| IBIS File
| Lattice Semiconductor Corporation
|[Doc Num]   FPGA-MD-02066 Ver. 1.0
[IBIS Ver]   4.2
[File name]   lifmd.ibs
[File rev]   2.5
[Date]   Mon May  6 22:10:33 PDT 2024
[Source]   Lattice Semiconductor umc40lp Process
[Notes]   Device: LIF-MD6000   Final
   Device: LIA-MD6000   Final
   Lattice Semiconductor has worked hard to ensure the
   models below are accurate and complete.  However, the
   data below was generated using simulation of the
   input/output model files for the silicon.  Therefore,
   the data below is for reference and initial design
   purposes only.
   Lattice Semiconductor grants permission to use this
   data for use in printed circuit design using this
   Lattice programmable logic device.  Other use of this
   code, including the selling or duplication of any
   portion is strictly prohibited.
|   NAMING CONVENTION
   The IBIS [Model] header is limited by the specification to a
   total of characters.  With such a set of characters available
   for naming models it becomes important to attempt to
   meaningfully encode the IO standards so they fit within the
   twenty character limit.  It would seem that twenty characters
   would provide room enough for describing IO's.  However, the
   PLD IO structure continues to grow more and more complex.  The
   complexity is making the twenty characters insuffiently
   descriptive.  In order to overcome this issue the naming
   convention described below is implemented to resolve the issue.
The twenty character space is managed as follows:
   bbbvvvsdddprtaaaoixx
   b = standard
   v = voltage (x.xx V)
   s = slew code
   d = drive (xx.x ma)
   p = pullmode code
   r = impedance
   t = mipi hard dphy mode
   o = diff resistor code
   i = diff  current code
   x = reserved
   standard
   LVCMOS   lvc
   lvcmosd   lvd
   LVTTL   lvt
   lvttld   ltd
   lvds   lvs
   sublvds   slv
   slvs   svs
   mipi   mip
   slew
   na   a
   fast   f
   slow   s
   pullmode
   off   a
   pull up   b
   3p3k   i
   6p8k   j
   10k   k
   impedance
   off   a
   mipi hard dphy mode
   off   a
   lp   l
   hs   h
   differential resistor
   off   a
   100   b
   differential current
   NA   a
   3.5   c
   Reserved   IO type
   in   input only (mipi: rx)
   ou   output (mipi: tx)
   io   I/O
   od   Open drain
   ic   Inverting differential input
   (signal name only)
   it   Non-Inverting differential
   input (signal name only)
   on   Inverting differential output
   (signal name only)
   op   Non-Inverting differential output
   (signal name only)
   bn   Inverting differential I/O
   (signal name only)
   bp   Non-Inverting differential I/O
   (signal name only)
   Lattice Semiconductor Corporation
   5555 NE Moore Court
   Hillsboro, OR 97214
   U.S.A
   TEL: 1-800-Lattice (USA and Canada)
   408-826-6000 (other locations)
   web: http://www.latticesemi.com/
   email: techsupport@latticesemi.com
The IBIS models by default includes the worst case package data
under [package].  If detailed package model is required , it can be
enable using [package model] keyword.
The .pkg files are included in the zip file with the IBIS models.
The .pkg file has to be located in the same directory as IBIS file.
[Disclaimer] This IBIS source code is intended as a design reference
   which illustrates how the Lattice Semiconductor device operates.
   It is the user's responsibility to verify their design for
   consistency and functionality through the use of formal
   verification methods.  Lattice Semiconductor provides no warranty
   regarding the use or functionality of this data.
[Copyright]   Copyright 2015 by Lattice Semiconductor Corporation
|   Component LIFMD
[Component]   LIFMD
[Manufacturer]   Lattice Semiconductor Corp.
[Package]
|CTFBGA80
| variable   typ   min   max
|R_pkg   144.360m   14.366m   221.160m
|L_pkg   1.9200nH   0.2595nH   2.6330nH
|C_pkg   0.3261pF   0.1794pF   1.7020pF
|CKFBGA80
| variable   typ   min   max
|R_pkg   164.7m   95.584m   220.49m
|L_pkg   1.53nH   0.8748nH   1.98nH
|C_pkg   0.7937pF   0.5599pF   0.9311pF
|CSFBGA81
| variable   typ   min   max
R_pkg   84.890m   15.155m   139.180m
L_pkg   1.1430nH   0.1667nH   1.6950nH
C_pkg   0.2490pF   0.1302pF   1.0720pF
|UCFBGA64
| variable   typ   min   max
|R_pkg   61.058m   18.526m   203.120m
|L_pkg   0.7464nH   0.1790nH   2.8510nH
|C_pkg   0.1780pF   0.1230pF   0.3352pF
|WLCSP36
| variable   typ   min   max
|R_pkg   291.220m   40.591m   563.790m
|L_pkg   0.5450nH   0.1240nH   1.7370nH
|C_pkg   0.2944pF   0.1749pF   0.3947pF
[Pin]  signal_name   model_name   R_pin   L_pin   C_pin
1   ltd330a080aaaaaaaaop   ltd330a080aaaaaaaaou
2   ltd330a080aaaaaaaaon   ltd330a080aaaaaaaaou
3   lvc120a020aaaaaaaaio   lvc120a020aaaaaaaaio
4   lvc120a020aaaaaaaaod   lvc120a020aaaaaaaaod
5   lvc120a020aaaaaaaaou   lvc120a020aaaaaaaaou
6   lvc120axxxaaaaaaaain   lvc120axxxaaaaaaaain
7   lvc120axxxbaaaaaaain   lvc120axxxbaaaaaaain
8   lvc180a040aaaaaaaaio   lvc180a040aaaaaaaaio
9   lvc180a040aaaaaaaaod   lvc180a040aaaaaaaaod
10   lvc180a040aaaaaaaaou   lvc180a040aaaaaaaaou
11   lvc180a040baaaaaaaio   lvc180a040baaaaaaaio
12   lvc180a040iaaaaaaaio   lvc180a040iaaaaaaaio
13   lvc180a040jaaaaaaaio   lvc180a040jaaaaaaaio
14   lvc180a040kaaaaaaaio   lvc180a040kaaaaaaaio
15   lvc180axxxaaaaaaaain   lvc180axxxaaaaaaaain
16   lvc180axxxbaaaaaaain   lvc180axxxbaaaaaaain
17   lvc180axxxiaaaaaaain   lvc180axxxiaaaaaaain
18   lvc180axxxjaaaaaaain   lvc180axxxjaaaaaaain
19   lvc180axxxkaaaaaaain   lvc180axxxkaaaaaaain
20   lvc250a060aaaaaaaaio   lvc250a060aaaaaaaaio
21   lvc250a060aaaaaaaaod   lvc250a060aaaaaaaaod
22   lvc250a060aaaaaaaaou   lvc250a060aaaaaaaaou
23   lvc250a060baaaaaaaio   lvc250a060baaaaaaaio
24   lvc250a060iaaaaaaaio   lvc250a060iaaaaaaaio
25   lvc250a060jaaaaaaaio   lvc250a060jaaaaaaaio
26   lvc250a060kaaaaaaaio   lvc250a060kaaaaaaaio
27   lvc250axxxaaaaaaaain   lvc250axxxaaaaaaaain
28   lvc250axxxbaaaaaaain   lvc250axxxbaaaaaaain
29   lvc250axxxiaaaaaaain   lvc250axxxiaaaaaaain
30   lvc250axxxjaaaaaaain   lvc250axxxjaaaaaaain
31   lvc250axxxkaaaaaaain   lvc250axxxkaaaaaaain
32   lvc330a080aaaaaaaaio   lvc330a080aaaaaaaaio
33   lvc330a080aaaaaaaaod   lvc330a080aaaaaaaaod
34   lvc330a080aaaaaaaaou   lvc330a080aaaaaaaaou
35   lvc330a080baaaaaaaio   lvc330a080baaaaaaaio
36   lvc330a080iaaaaaaaio   lvc330a080iaaaaaaaio
37   lvc330a080jaaaaaaaio   lvc330a080jaaaaaaaio
38   lvc330a080kaaaaaaaio   lvc330a080kaaaaaaaio
39   lvc330axxxaaaaaaaain   lvc330axxxaaaaaaaain
40   lvc330axxxbaaaaaaain   lvc330axxxbaaaaaaain
41   lvc330axxxiaaaaaaain   lvc330axxxiaaaaaaain
42   lvc330axxxjaaaaaaain   lvc330axxxjaaaaaaain
43   lvc330axxxkaaaaaaain   lvc330axxxkaaaaaaain
44   lvd250a060aaaaaaaabp   lvd250a060aaaaaaaaio
45   lvd250a060aaaaaaaabn   lvd250a060aaaaaaaaio
46   lvd250a060aaaaaaaaop   lvd250a060aaaaaaaaou
47   lvd250a060aaaaaaaaon   lvd250a060aaaaaaaaou
48   lvd250axxxaaaaaaaait   lvd250axxxaaaaaaaain
49   lvd250axxxaaaaaaaaic   lvd250axxxaaaaaaaain
50   lvd330a080aaaaaaaaop   lvd330a080aaaaaaaaou
51   lvd330a080aaaaaaaaon   lvd330a080aaaaaaaaou
52   lvs250axxxaaaaaaaait   lvs250axxxaaaaaaaain
53   lvs250axxxaaaaaaaaic   lvs250axxxaaaaaaaain
54   lvs250axxxaaaaaaacop   lvs250axxxaaaaaaacou
55   lvs250axxxaaaaaaacon   lvs250axxxaaaaaaacou
56   lvs250axxxaaaaaabait   lvs250axxxaaaaaabain
57   lvs250axxxaaaaaabaic   lvs250axxxaaaaaabain
58   lvt330a080aaaaaaaaio   lvt330a080aaaaaaaaio
59   lvt330a080aaaaaaaaod   lvt330a080aaaaaaaaod
60   lvt330a080aaaaaaaaou   lvt330a080aaaaaaaaou
61   lvt330a080baaaaaaaio   lvt330a080baaaaaaaio
62   lvt330a080iaaaaaaaio   lvt330a080iaaaaaaaio
63   lvt330a080jaaaaaaaio   lvt330a080jaaaaaaaio
64   lvt330a080kaaaaaaaio   lvt330a080kaaaaaaaio
65   lvt330axxxaaaaaaaain   lvt330axxxaaaaaaaain
66   lvt330axxxbaaaaaaain   lvt330axxxbaaaaaaain
67   lvt330axxxiaaaaaaain   lvt330axxxiaaaaaaain
68   lvt330axxxjaaaaaaain   lvt330axxxjaaaaaaain
69   lvt330axxxkaaaaaaain   lvt330axxxkaaaaaaain
70   mip120a020aaaaaaaabp   mip120a020aaaaaaaaio
71   mip120a020aaaaaaaabn   mip120a020aaaaaaaaio
72   mip120axxxaaaaaabait   mip120axxxaaaaaabain
73   mip120axxxaaaaaabaic   mip120axxxaaaaaabain
74   mip120a020aaaaaaaaop   mip120a020aaaaaaaaou
75   mip120a020aaaaaaaaon   mip120a020aaaaaaaaou
76   mip120axxxaaaaaaaait   mip120axxxaaaaaaaain
77   mip120axxxaaaaaaaaic   mip120axxxaaaaaaaain
78   slv250axxxaaaaaaaait   slv250axxxaaaaaaaain
79   slv250axxxaaaaaaaaic   slv250axxxaaaaaaaain
80   slv250axxxaaaaaabait   slv250axxxaaaaaabain
81   slv250axxxaaaaaabaic   slv250axxxaaaaaabain
82   svs120axxxaaaaaaaait   svs120axxxaaaaaaaain
83   svs120axxxaaaaaaaaic   svs120axxxaaaaaaaain
84   svs120axxxaaaaaabait   svs120axxxaaaaaabain
85   svs120axxxaaaaaabaic   svs120axxxaaaaaabain
86   mip120axxxaahaaaaait   mip120axxxaahaaaaain
87   mip120axxxaahaaaaaic   mip120axxxaahaaaaain
88   mip120axxxaahaaaaaop   mip120axxxaahaaaaaou
89   mip120axxxaahaaaaaon   mip120axxxaahaaaaaou
90   mip120axxxaalaaaaain   mip120axxxaalaaaaain
91   mip120axxxaalaaaaaou   mip120axxxaalaaaaaou
92   GND   GND
93   POWER   POWER
[Diff pin]  inv_pin  vdiff  tdelay_typ  tdelay_min  tdelay_max
1   2   0.1   0.0s   0.0s   0.0s
44   45   NA   NA   NA   NA
46   47   0.1   0.0s   0.0s   0.0s
48   49   NA   NA   NA   NA
50   51   0.1   0.0s   0.0s   0.0s
52   53   NA   NA   NA   NA
54   55   0.1   0.0s   0.0s   0.0s
56   57   NA   NA   NA   NA
70   71   NA   NA   NA   NA
72   73   NA   NA   NA   NA
74   75   NA   NA   NA   NA
76   77   NA   NA   NA   NA
78   79   NA   NA   NA   NA
80   81   NA   NA   NA   NA
82   83   NA   NA   NA   NA
84   85   NA   NA   NA   NA
86   87   NA   NA   NA   NA
88   89   0.1   0.0s   0.0s   0.0s
[Series Pin Mapping]  pin_2   model_name   function_table_group
56   57   lvss
72   73   lvss
80   81   lvss
84   85   lvss
[Model]  lvss
Model_type   Series
C_comp   0  0  0
[Voltage Range]  2.50V   2.38V   2.63V
[R Series]   100   110   90
|End [Model]
|End [Component]
| Models and submodels in the file (74): ltd330a080aaaaaaaaou (Output), lvc120a020aaaaaaaaio (I/O), lvc120a020aaaaaaaaod (I/O_open_drain), lvc120axxxaaaaaaaain (Input), lvc120axxxbaaaaaaain (Input), lvc120a020aaaaaaaaou (Output), lvc180a040aaaaaaaaio (I/O), lvc180a040aaaaaaaaod (I/O_open_drain), lvc180a040aaaaaaaaou (Output), lvc180a040baaaaaaaio (I/O), lvc180a040iaaaaaaaio (I/O), lvc180a040jaaaaaaaio (I/O), lvc180a040kaaaaaaaio (I/O), lvc180axxxaaaaaaaain (Input), lvc180axxxbaaaaaaain (Input), lvc180axxxiaaaaaaain (Input), lvc180axxxjaaaaaaain (Input), lvc180axxxkaaaaaaain (Input), lvc250a060aaaaaaaaio (I/O), lvc250a060aaaaaaaaod (I/O_open_drain), lvc250a060aaaaaaaaou (Output), lvc250a060baaaaaaaio (I/O), lvc250a060iaaaaaaaio (I/O), lvc250a060jaaaaaaaio (I/O), lvc250a060kaaaaaaaio (I/O), lvc250axxxaaaaaaaain (Input), lvc250axxxbaaaaaaain (Input), lvc250axxxiaaaaaaain (Input), lvc250axxxjaaaaaaain (Input), lvc250axxxkaaaaaaain (Input), lvc330a080aaaaaaaaio (I/O), lvc330a080aaaaaaaaod (I/O_open_drain), lvc330a080aaaaaaaaou (Output), lvc330a080baaaaaaaio (I/O), lvc330a080iaaaaaaaio (I/O), lvc330a080jaaaaaaaio (I/O), lvc330a080kaaaaaaaio (I/O), lvc330axxxaaaaaaaain (Input), lvc330axxxbaaaaaaain (Input), lvc330axxxiaaaaaaain (Input), lvc330axxxjaaaaaaain (Input), lvc330axxxkaaaaaaain (Input), lvd250a060aaaaaaaaio (I/O), lvd250a060aaaaaaaaou (Output), lvd250axxxaaaaaaaain (Input), lvd330a080aaaaaaaaou (Output), lvs250axxxaaaaaaaain (Input), lvs250axxxaaaaaaacou (Output), lvs250axxxaaaaaabain (Input), lvt330a080aaaaaaaaio (I/O), lvt330a080aaaaaaaaod (I/O_open_drain), lvt330a080aaaaaaaaou (Output), lvt330a080baaaaaaaio (I/O), lvt330a080iaaaaaaaio (I/O), lvt330a080jaaaaaaaio (I/O), lvt330a080kaaaaaaaio (I/O), lvt330axxxaaaaaaaain (Input), lvt330axxxbaaaaaaain (Input), lvt330axxxiaaaaaaain (Input), lvt330axxxjaaaaaaain (Input), lvt330axxxkaaaaaaain (Input), mip120a020aaaaaaaaio (I/O), mip120axxxaaaaaabain (Input), mip120a020aaaaaaaaou (Output), mip120axxxaaaaaaaain (Input), slv250axxxaaaaaaaain (Input), slv250axxxaaaaaabain (Input), svs120axxxaaaaaaaain (Input), svs120axxxaaaaaabain (Input), mip120axxxaahaaaaain (Input), mip120axxxaahaaaaaou (Output), mip120axxxaalaaaaain (Input), mip120axxxaalaaaaaou (Output), lvss (Series)
